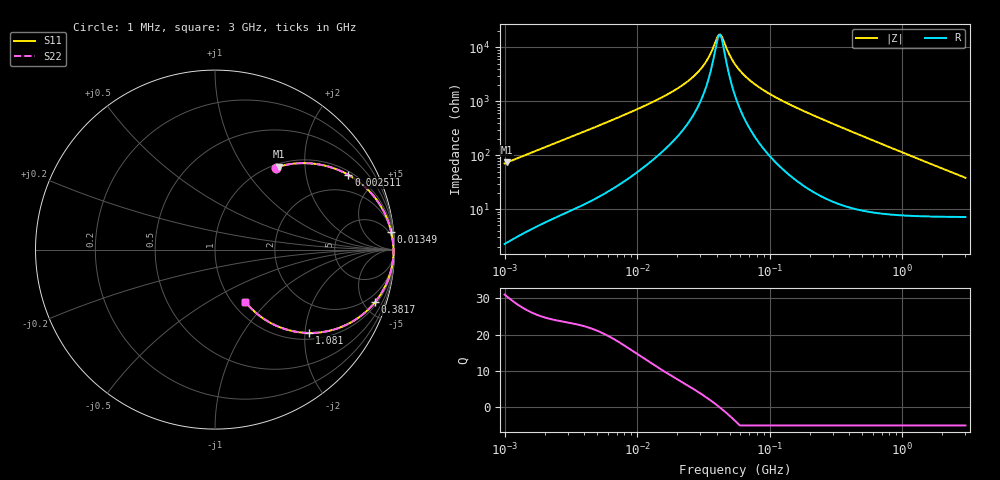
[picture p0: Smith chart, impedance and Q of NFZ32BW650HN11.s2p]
! NFZ32BW650HN11
# Hz S RI R 50
!Freq.(Hz) S11(Real) S11(Imag) S21(Real) S21(Imag) S12(Real) S12(Imag) S22(Real) S22(Imag)
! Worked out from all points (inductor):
!   401 points, 1 MHz to 3 GHz, reference 50 ohm
!   read as one part in series: L = 11.2 uH near 1.041 MHz
!   highest Q = 30.5 at 1.041 MHz (marker M1), where L = 11.2 uH
!   self-resonance near 41.39 MHz
!   S11 on the Smith chart (normalised r, x): 1 MHz: 1.05, +1.41; 2.511 MHz: 1.15, +3.48; 13.49 MHz: 3, +20; 381.7 MHz: 1.22, -5.99; 1.081 GHz: 1.15, -2.09; 3 GHz: 1.14, -0.75
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1000000  0.3381 0.4572  0.6619 -0.4572  0.6619 -0.4572  0.3381 0.4572
1040844  0.3554 0.4625  0.6446 -0.4625  0.6446 -0.4625  0.3554 0.4625
1584654  0.5498 0.4788  0.4502 -0.4788  0.4502 -0.4788  0.5498 0.4788
2511129  0.743 0.4166  0.257 -0.4166  0.257 -0.4166  0.743 0.4166
3823119  0.8636 0.3218  0.1364 -0.3218  0.1364 -0.3218  0.8636 0.3218
1.349163e7  0.9821 0.0963  0.0179 -0.0963  0.0179 -0.0963  0.9821 0.0963
1.461624e7  0.984 0.0875  0.016 -0.0875  0.016 -0.0875  0.984 0.0875
2.137957e7  0.9901 0.0512  0.00989 -0.0512  0.00989 -0.0512  0.9901 0.0512
2.829425e7  0.9926 0.0288  0.00738 -0.0288  0.00738 -0.0288  0.9926 0.0288
3.387922e7  0.9936 0.0154  0.00638 -0.0154  0.00638 -0.0154  0.9936 0.0154
4.138676e7  0.9943 0.000981  0.00574 -0.000981  0.00574 -0.000981  0.9943 0.000981
4.394807e7  0.9944 -0.00336  0.00565 0.00336  0.00565 0.00336  0.9944 -0.00336
4.955604e7  0.9944 -0.0121  0.0056 0.0121  0.0056 0.0121  0.9944 -0.0121
5.477226e7  0.9943 -0.0196  0.00571 0.0196  0.00571 0.0196  0.9943 -0.0196
6.690963e7  0.9936 -0.0352  0.0064 0.0352  0.0064 0.0352  0.9936 -0.0352
8.679508e7  0.9916 -0.0577  0.00844 0.0577  0.00844 0.0577  0.9916 -0.0577
2.094008e8  0.9633 -0.1699  0.0367 0.1699  0.0367 0.1699  0.9633 -0.1699
3.817355e8  0.8912 -0.2933  0.1088 0.2933  0.1088 0.2933  0.8912 -0.2933
8.005644e8  0.6593 -0.4465  0.3407 0.4465  0.3407 0.4465  0.6593 -0.4465
1.080907e9  0.5227 -0.4645  0.4773 0.4645  0.4773 0.4645  0.5227 -0.4645
1.855641e9  0.2952 -0.4003  0.7048 0.4003  0.7048 0.4003  0.2952 -0.4003
3e9  0.1696 -0.292  0.8304 0.292  0.8304 0.292  0.1696 -0.292
